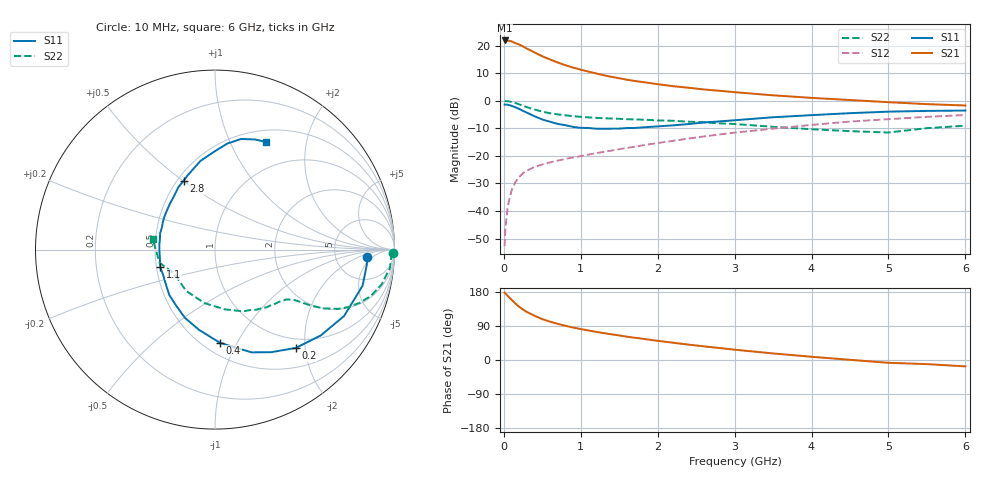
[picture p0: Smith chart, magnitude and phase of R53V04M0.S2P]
! SIEMENS Small Signal Semiconductors
! BFR183
! Si NPN RF Bipolar Junction Transistor in SOT23
! VCE = 3 V  IC = 4 mA
! Common Emitter S-Parameters:  May  1996
# GHz  S  MA  R  50
!  f  S11  S21  S12  S22
! GHz  MAG  ANG  MAG  ANG  MAG  ANG  MAG  ANG
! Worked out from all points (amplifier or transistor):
!   36 points, 10 MHz to 6 GHz, reference 50 ohm
!   highest |S21| = 21.9 dB at 10 MHz (marker M1)
!   |S21| within 3 dB of that: start of sweep to 301.7 MHz
!   unconditionally stable (mu >= 1): 1.138 GHz to 2.655 GHz
!   at 250 MHz: K = 0.37, MSG = 23.0 dB, |S12| = -26.3 dB
!   at 1.4 GHz: K = 1.06, MAG = 11.9 dB, |S12| = -18.1 dB
!   at 6 GHz: K = 0.89, MSG = 1.7 dB, |S12| = -5.2 dB
!   S11 on the Smith chart (normalised r, x): 10 MHz: 11, -4; 200 MHz: 0.83, -1.82; 400 MHz: 0.60, -0.86; 1.1 GHz: 0.52, -0.11; 2.8 GHz: 0.54, +0.50; 6 GHz: 0.64, +1.37
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0.01  0.8507 -2.9  12.38 178.0  0.0023 87.8  0.993 -1.2
0.02  0.85 -5.7  12.21 175.5  0.0048 87.6  0.9826 -2.4
0.05  0.8466 -13.7  12.22 169.3  0.0119 81.7  0.9801 -6.0
0.1  0.8089 -27.2  11.93 159.1  0.0233 76.6  0.949 -11.7
0.15  0.7588 -39.1  11.07 149.0  0.0335 69.6  0.9068 -16.5
0.2  0.7095 -50.5  10.45 140.5  0.0416 65.9  0.8589 -20.2
0.25  0.6522 -61.2  9.642 132.8  0.0485 61.5  0.807 -23.4
0.3  0.6077 -70.4  8.791 126.7  0.0539 58.8  0.7642 -25.6
0.4  0.5208 -86.8  7.499 116.7  0.0631 55.0  0.6914 -28.3
0.5  0.4566 -101.1  6.409 107.8  0.0698 53.3  0.633 -29.9
0.6  0.4156 -113.8  5.601 101.2  0.0761 52.7  0.5921 -30.8
0.7  0.3802 -124.5  4.937 95.4  0.0819 52.6  0.5651 -31.4
0.9  0.3352 -144.7  3.989 85.7  0.0936 53.2  0.5247 -32.4
1.1  0.3204 -162.7  3.373 77.9  0.1056 54.7  0.4987 -33.9
1.3  0.3098 -177.9  2.897 70.9  0.1183 55.6  0.4815 -35.4
1.6  0.3193 163.2  2.401 61.5  0.1392 56.6  0.4629 -38.8
2.2  0.3574 134.9  1.833 45.6  0.1875 56.3  0.4323 -47.9
2.8  0.4212 114.6  1.515 31.7  0.2442 53.0  0.3887 -60.2
3.5  0.5013 99.2  1.252 17.3  0.3115 46.3  0.3366 -81.0
4.5  0.5946 83.4  1.03 0.5  0.4187 34.5  0.2805 -125.0
5.5  0.6529 70.0  0.867 -10.9  0.5096 21.7  0.3177 -166.7
6  0.6632 64.7  0.819 -16.8  0.5508 13.2  0.3522 170.2
